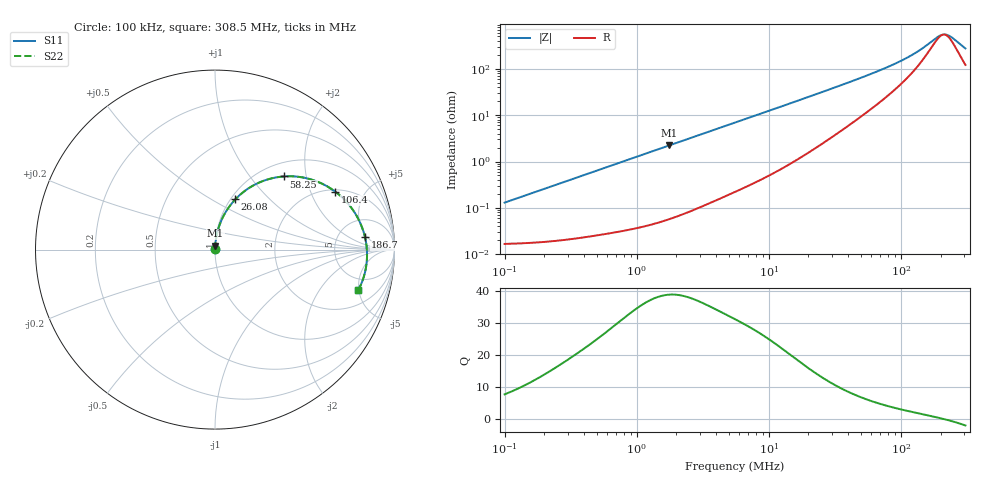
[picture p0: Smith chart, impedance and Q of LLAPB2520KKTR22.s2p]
! LLAPB2520KKTR22  S-PARAMETER MODEL  ( General Type )
! Model Generated by TAIYO YUDEN Corporation (http://www.ty-top.com)
! Version 2.0
! TAIYO YUDEN Control No. 20210629
! Copyright(c) 2015 TAIYO YUDEN CO.,LTD. All Rights Reserved.
! Product Description (link to TY-COMPAS)
! https://ds.yuden.co.jp/TYCOMPAS/or/detail?pn=LLAPB2520KKTR22M&u=M
! Products Name : Inductors
! Characteristics :
!  Inductance : 0.22 uH , SRF(min) : -Hz , DC Resistance(max) : 0.021 Ohm
!  Rated Current : Saturation :7500 mA , Temp Rise : 4900 mA (40 degC)
!  Case Size : 2.5 x 2.0 / 0.098 x 0.079 [mm/inch] , Thickness : 1 / 0.039 [mm/inch]
!  (Conditions: Temperature = 25 degC , DC Bias Current/Voltage = 0A / 0V)
! External Node Assignments :
!  1  o---GGG---o  2
! GND o---------o GND
! Frequency Range : 0.1MHz  -  308.54851MHz  [ 402 STEP ]
# MHz S RI R 50
! Freq[MHz].  S11 Real  S11 Imag  S21 Real  S21 Imag  S12 Real  S12 Imag  S22 Real  S22 Imag
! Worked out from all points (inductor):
!   401 points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, 100 kHz to 308.5 MHz, reference 50 ohm
!   read as one part in series: L = 205 nH near 104.1 kHz
!   highest Q = 39 at 1.768 MHz (marker M1), where L = 200 nH
!   self-resonance near 211 MHz
!   S11 on the Smith chart (normalised r, x): 100 kHz: 1.00, +0.00; 26.08 MHz: 1.05, +0.65; 58.25 MHz: 1.26, +1.50; 106.4 MHz: 2.10, +3.04; 186.7 MHz: 9, +4; 308.5 MHz: 3.44, -4.95
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0.1  0.000168 0.00129  0.9998 -0.00129  0.9998 -0.00129  0.000168 0.00129
0.384115  0.000251 0.0049  0.9997 -0.0049  0.9997 -0.0049  0.000251 0.0049
1.475446  0.000829 0.0186  0.9992 -0.0186  0.9992 -0.0186  0.000829 0.0186
1.7678  0.00106 0.0222  0.9989 -0.0222  0.9989 -0.0222  0.00106 0.0222
5.667415  0.00716 0.0698  0.9928 -0.0698  0.9928 -0.0698  0.00716 0.0698
11.2196  0.0244 0.1345  0.9756 -0.1345  0.9756 -0.1345  0.0244 0.1345
15.78606  0.0457 0.1842  0.9543 -0.1842  0.9543 -0.1842  0.0457 0.1842
21.33651  0.0792 0.239  0.9208 -0.239  0.9208 -0.239  0.0792 0.239
26.08294  0.1131 0.2799  0.8869 -0.2799  0.8869 -0.2799  0.1131 0.2799
38.97828  0.22 0.3609  0.78 -0.3609  0.78 -0.3609  0.22 0.3609
48.61598  0.304 0.3941  0.696 -0.3941  0.696 -0.3941  0.304 0.3941
58.24905  0.3846 0.4077  0.6154 -0.4077  0.6154 -0.4077  0.3846 0.4077
69.79087  0.4718 0.4047  0.5282 -0.4047  0.5282 -0.4047  0.4718 0.4047
81.95682  0.5508 0.3859  0.4492 -0.3859  0.4492 -0.3859  0.5508 0.3859
106.4114  0.671 0.3221  0.329 -0.3221  0.329 -0.3221  0.671 0.3221
138.1628  0.768 0.2215  0.232 -0.2215  0.232 -0.2215  0.768 0.2215
186.7415  0.8358 0.0696  0.1642 -0.0696  0.1642 -0.0696  0.8358 0.0696
206.4702  0.8452 0.0126  0.1548 -0.0126  0.1548 -0.0126  0.8452 0.0126
223.7435  0.8472 -0.0345  0.1528 0.0345  0.1528 0.0345  0.8472 -0.0345
242.462  0.8438 -0.0824  0.1562 0.0824  0.1562 0.0824  0.8438 -0.0824
296.3991  0.8102 -0.2013  0.1898 0.2013  0.1898 0.2013  0.8102 -0.2013
308.5485  0.7991 -0.224  0.2009 0.224  0.2009 0.224  0.7991 -0.224
